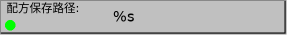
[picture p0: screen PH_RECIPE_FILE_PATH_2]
VISUALIZATION PH_RECIPE_FILE_PATH_2  // 287x35
VAR_INPUT
	RECIPE_CTRL_V2 : ST_RecipeCtrl_2;
END_VAR
VAR_INPUT
	Right_Edge_Rel : UDINT;
END_VAR
    Rectangle (0,0 285x33), "配方保存路径:", input disabled if: TRUE, text list: 'TextList_Recipe', text index: 100
        p874137650: Right_Edge_Rel
    Rectangle (110,0 175x33), "%s", text variable: RECIPE_CTRL_V2.sStatus.sgFilePath
        p874137650: Right_Edge_Rel
    Ellipse (5,20 10x10), invisible if: NOT RECIPE_CTRL_V2.sStatus.bInitialOk
END_VISUALIZATION
